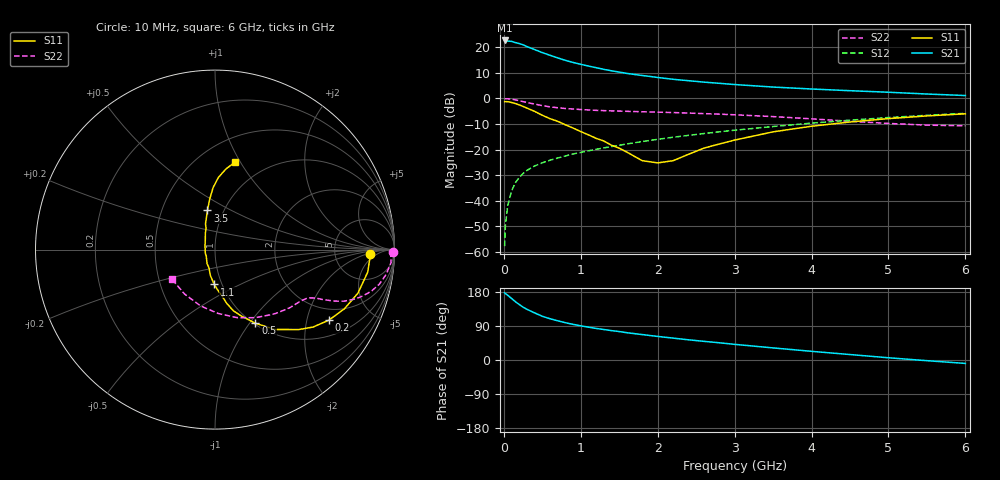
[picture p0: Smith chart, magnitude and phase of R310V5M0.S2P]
! SIEMENS Small Signal Semiconductors
! BFR181
! Si NPN RF Bipolar Junction Transistor in SOT23
! VCE = 10 V  IC = 5 mA
! Common Emitter S-Parameters:  May  1996
# GHz  S  MA  R  50
!  f  S11  S21  S12  S22
! GHz  MAG  ANG  MAG  ANG  MAG  ANG  MAG  ANG
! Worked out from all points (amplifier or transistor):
!   36 points, 10 MHz to 6 GHz, reference 50 ohm
!   highest |S21| = 22.6 dB at 10 MHz (marker M1)
!   |S21| within 3 dB of that: start of sweep to 353.3 MHz
!   unconditionally stable (mu >= 1): 1.219 GHz to 3.157 GHz
!   at 250 MHz: K = 0.41, MSG = 25.1 dB, |S12| = -29.3 dB
!   at 1.4 GHz: K = 1.03, MAG = 13.7 dB, |S12| = -18.8 dB
!   at 6 GHz: K = 0.87, MSG = 3.5 dB, |S12| = -5.8 dB
!   S11 on the Smith chart (normalised r, x): 10 MHz: 13, -3; 200 MHz: 1.54, -2.73; 500 MHz: 1.02, -1.07; 1.1 GHz: 0.92, -0.37; 3.5 GHz: 0.84, +0.38; 6 GHz: 0.73, +0.95
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0.01  0.8655 -1.7  13.52 177.2  0.0013 91.3  0.9909 -0.8
0.02  0.8638 -3.5  13.17 175.5  0.0033 86.1  0.9795 -1.7
0.05  0.86 -8.4  13.16 170.9  0.008 82.9  0.9834 -4.2
0.1  0.8327 -16.9  12.98 162.5  0.0155 82.0  0.964 -8.2
0.15  0.7927 -24.6  12.28 153.8  0.0225 76.8  0.9355 -11.9
0.2  0.7464 -31.8  11.78 146.5  0.0286 73.3  0.9025 -14.8
0.25  0.6962 -38.3  11.11 139.5  0.0341 70.2  0.865 -17.3
0.3  0.6459 -43.6  10.29 133.8  0.0392 68.7  0.831 -19.3
0.4  0.5575 -53.0  8.983 124.3  0.0479 65.8  0.7738 -21.8
0.5  0.4681 -61.2  7.828 115.4  0.0551 64.3  0.723 -23.4
0.6  0.4014 -68.0  6.943 108.9  0.062 63.8  0.6833 -24.3
0.8  0.3046 -77.9  5.526 98.5  0.0751 63.3  0.6343 -25.4
0.9  0.2633 -81.1  5.026 94.0  0.0822 63.3  0.6197 -25.9
1.1  0.1939 -91.2  4.281 86.7  0.0946 64.0  0.5943 -26.9
1.3  0.147 -100.0  3.687 80.5  0.1079 63.8  0.576 -28.3
1.6  0.0893 -119.9  3.075 72.0  0.1291 63.5  0.5587 -30.8
1.8  0.0606 -143.4  2.797 67.1  0.1436 63.1  0.5481 -32.8
2.2  0.0607 156.1  2.358 57.8  0.1741 61.7  0.5287 -37.6
3.5  0.222 100.9  1.663 31.9  0.2822 53.0  0.4408 -59.4
4.5  0.3462 91.7  1.412 14.4  0.3755 43.1  0.3567 -87.0
5.5  0.4543 82.2  1.216 -1.8  0.4673 31.1  0.3001 -124.3
6  0.4995 77.1  1.136 -9.0  0.5107 24.5  0.2914 -145.4
